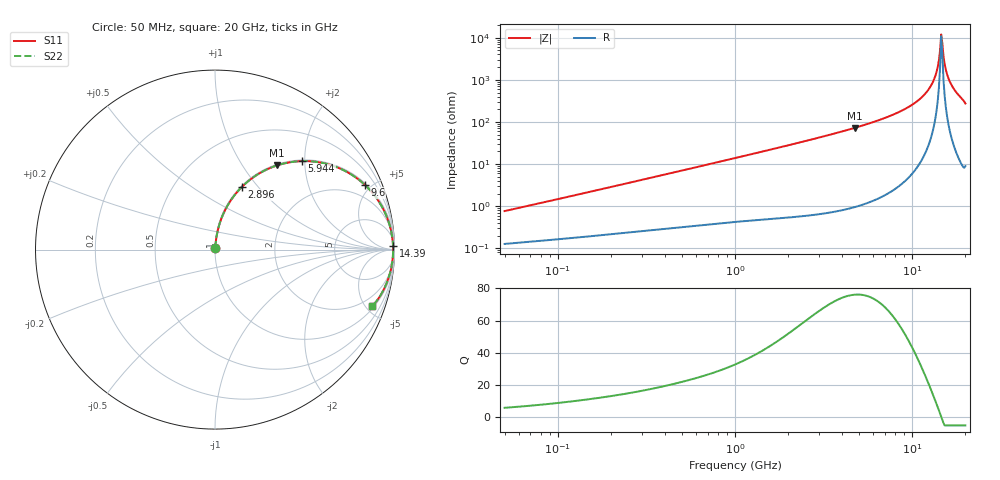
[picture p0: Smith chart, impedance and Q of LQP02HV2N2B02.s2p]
!Murata Part Number: LQP02HV2N2B02
!These Parameters are Measured in Series Mode Connection
!  o--[Z]--o
!Port1  Port2
!  o-------o
!Freq. Start=50[MHz] Stop=20[GHz], 401[Steps]
# Hz S RI R 50
!Freq.(Hz) S11(Real) S11(Imag) S21(Real) S21(Imag) S12(Real) S12(Imag) S22(Real) S22(Imag)
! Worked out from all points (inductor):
!   401 points, 50 MHz to 20 GHz, reference 50 ohm
!   read as one part in series: L = 2.38 nH near 51.52 MHz
!   highest Q = 76.1 at 4.748 GHz (marker M1), where L = 2.43 nH
!   self-resonance near 14.6 GHz
!   S11 on the Smith chart (normalised r, x): 50 MHz: 1.00, +0.02; 2.896 GHz: 1.01, +0.82; 5.944 GHz: 1.03, +1.94; 9.6 GHz: 1.10, +4.58; 14.39 GHz: open; 20 GHz: 1.18, -5.48
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5e7  0.00133 0.00754  0.9987 -0.00754  0.9987 -0.00754  0.00133 0.00754
1.364002e8  0.00223 0.0197  0.9978 -0.0197  0.9978 -0.0197  0.00223 0.0197
3.721004e8  0.00551 0.0519  0.9945 -0.0519  0.9945 -0.0519  0.00551 0.0519
1e9  0.0228 0.1349  0.9772 -0.1349  0.9772 -0.1349  0.0228 0.1349
2.728004e9  0.134 0.3328  0.866 -0.3328  0.866 -0.3328  0.134 0.3328
2.896447e9  0.1492 0.3486  0.8508 -0.3486  0.8508 -0.3486  0.1492 0.3486
4.748272e9  0.3464 0.4693  0.6536 -0.4693  0.6536 -0.4693  0.3464 0.4693
5.944466e9  0.4858 0.4931  0.5142 -0.4931  0.5142 -0.4931  0.4858 0.4931
7.442007e9  0.6498 0.4694  0.3502 -0.4694  0.3502 -0.4694  0.6498 0.4694
9.600142e9  0.835 0.3607  0.165 -0.3607  0.165 -0.3607  0.835 0.3607
1.131968e10  0.9291 0.241  0.0709 -0.241  0.0709 -0.241  0.9291 0.241
1.276073e10  0.9735 0.1345  0.0265 -0.1345  0.0265 -0.1345  0.9735 0.1345
1.334722e10  0.9837 0.0916  0.0163 -0.0916  0.0163 -0.0916  0.9837 0.0916
1.375312e10  0.9883 0.0625  0.0117 -0.0625  0.0117 -0.0625  0.9883 0.0625
1.438523e10  0.9921 0.0183  0.00793 -0.0183  0.00793 -0.0183  0.9921 0.0183
1.482269e10  0.9923 -0.0114  0.00765 0.0114  0.00765 0.0114  0.9923 -0.0114
1.504638e10  0.9918 -0.0262  0.00818 0.0262  0.00818 0.0262  0.9918 -0.0262
1.550395e10  0.9894 -0.0559  0.0106 0.0559  0.0106 0.0559  0.9894 -0.0559
1.573793e10  0.9875 -0.0707  0.0125 0.0707  0.0125 0.0707  0.9875 -0.0707
1.646126e10  0.9793 -0.1147  0.0207 0.1147  0.0207 0.1147  0.9793 -0.1147
1.774144e10  0.9565 -0.1863  0.0435 0.1863  0.0435 0.1863  0.9565 -0.1863
2e10  0.8746 -0.3152  0.1254 0.3152  0.1254 0.3152  0.8746 -0.3152
